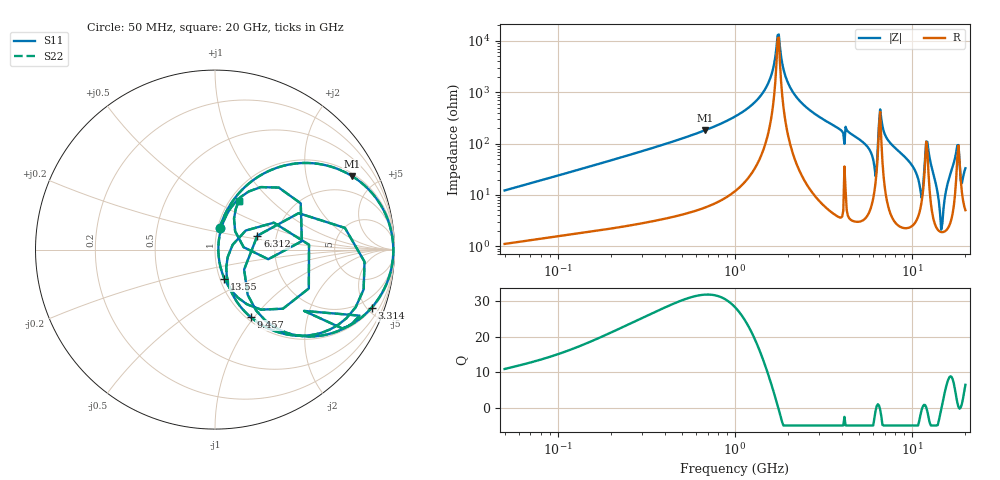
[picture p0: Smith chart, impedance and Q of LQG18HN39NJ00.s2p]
!Murata Part Number: LQG18HN39NJ00
!These Parameters are Measured in Series Mode Connection
!  o--[Z]--o
!Port1  Port2
!  o-------o
!Freq. Start=50[MHz] Stop=20[GHz], 401[Steps]
# Hz S RI R 50
!Freq.(Hz) S11(Real) S11(Imag) S21(Real) S21(Imag) S12(Real) S12(Imag) S22(Real) S22(Imag)
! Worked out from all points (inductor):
!   401 points, 50 MHz to 20 GHz, reference 50 ohm
!   read as one part in series: L = 38.5 nH near 51.52 MHz
!   highest Q = 31.9 at 677.4 MHz (marker M1), where L = 42.8 nH
!   self-resonance near 1.741 GHz
!   S11 on the Smith chart (normalised r, x): 50 MHz: 1.02, +0.24; 3.314 GHz: 1.11, -5.34; 6.312 GHz: 1.59, +0.26; 9.457 GHz: 1.05, -0.96; 13.55 GHz: 1.05, -0.35; 20 GHz: 1.10, +0.66
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5e7  0.0253 0.1177  0.9747 -0.1177  0.9747 -0.1177  0.0253 0.1177
1.364002e8  0.1081 0.2834  0.8919 -0.2834  0.8919 -0.2834  0.1081 0.2834
3.721004e8  0.4495 0.4796  0.5505 -0.4796  0.5505 -0.4796  0.4495 0.4796
6.774326e8  0.7614 0.4109  0.2386 -0.4109  0.2386 -0.4109  0.7614 0.4109
1e9  0.9109 0.2678  0.0891 -0.2678  0.0891 -0.2678  0.9109 0.2678
1.476162e9  0.9853 0.0861  0.0147 -0.0861  0.0147 -0.0861  0.9853 0.0861
1.766834e9  0.9934 -0.00356  0.00656 0.00356  0.00656 0.00356  0.9934 -0.00356
2.021818e9  0.9885 -0.072  0.0115 0.072  0.0115 0.072  0.9885 -0.072
2.728004e9  0.9392 -0.2258  0.0608 0.2258  0.0608 0.2258  0.9392 -0.2258
3.314454e9  0.872 -0.3241  0.128 0.3241  0.128 0.3241  0.872 -0.3241
5.598765e9  0.4331 -0.4731  0.5669 0.4731  0.5669 0.4731  0.4331 -0.4731
6.311513e9  0.2359 0.0773  0.7641 -0.0773  0.7641 -0.0773  0.2359 0.0773
6.701223e9  0.8281 -0.2222  0.1719 0.2222  0.1719 0.2222  0.8281 -0.2222
7.442007e9  0.5362 -0.4761  0.4638 0.4761  0.4638 0.4761  0.5362 -0.4761
9.457416e9  0.1984 -0.3757  0.8016 0.3757  0.8016 0.3757  0.1984 -0.3757
1.115139e10  0.0629 -0.0983  0.9371 0.0983  0.9371 0.0983  0.0629 -0.0983
1.238412e10  0.3785 -0.3294  0.6215 0.3294  0.6215 0.3294  0.3785 -0.3294
1.354865e10  0.0526 -0.1619  0.9474 0.1619  0.9474 0.1619  0.0526 -0.1619
1.460232e10  0.0188 -0.00898  0.9812 0.00898  0.9812 0.00898  0.0188 -0.00898
1.747767e10  0.2556 0.3483  0.7444 -0.3483  0.7444 -0.3483  0.2556 0.3483
1.88369e10  0.1596 0.0132  0.8404 -0.0132  0.8404 -0.0132  0.1596 0.0132
2e10  0.1331 0.2711  0.8669 -0.2711  0.8669 -0.2711  0.1331 0.2711
